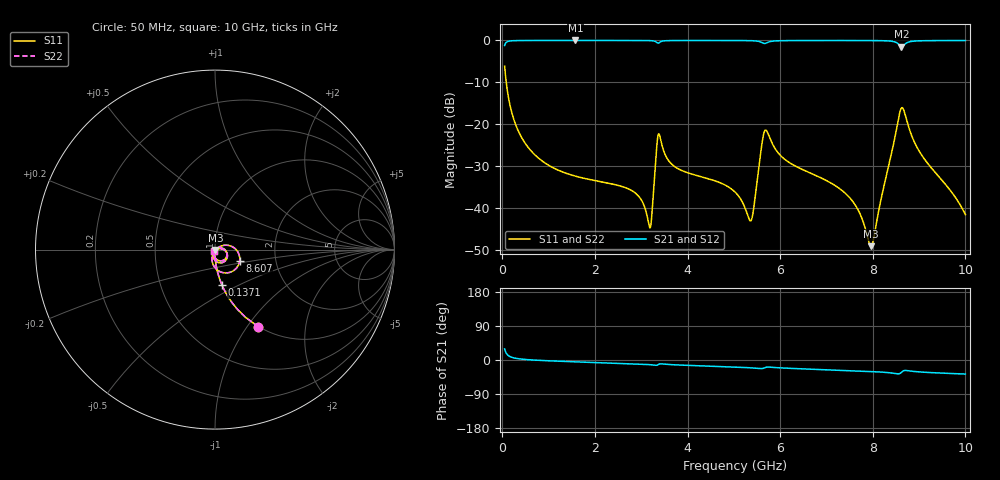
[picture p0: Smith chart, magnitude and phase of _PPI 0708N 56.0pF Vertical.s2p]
! S-Parameter data specifications (vertical orientation):
! Substrate: 40-mil Rogers 3003C, Substrate thickness, H=1.016mm, Dielectric constant, Er=3, Conductor thickness, T_mtl=0.043mm, Loss Tangent, Tand=0.003
! PCB Mounting Pad Footprint: Pad width, PadW=2.54mm , Pad length, PadL=0.51mm , Pad gap, PadG (edge-to-edge)=0.71mm , Reference planes=1.73mm apart
! Created Tue Jan 16 08:53:47 2018
# GHz S MA R 50
! 2 Port Network Data from SP1.SP block
! freq  magS11  angS11  magS21  angS21  magS12  angS12  magS22  angS22
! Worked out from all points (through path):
!   801 points, 50 MHz to 10 GHz, reference 50 ohm
!   highest |S21| = -0.01 dB at 1.58 GHz (marker M1); lowest = -1.5 dB at 8.619 GHz (marker M2)
!   group delay of S21, straight-line fit = 11.2 ps
!   lowest |S11| = -49.1 dB at 7.96 GHz (marker M3), VSWR 1.01, Z = 50.3 - j0.233 ohm
!   |S11| at or under -10 dB: 85.18 MHz to end of sweep
!   |S22| runs from -49.1 to -6.1 dB; largest |S21 - S12| = 0
!   S11 on the Smith chart (normalised r, x): 50 MHz: 1.00, -1.13; 137.1 MHz: 1.00, -0.41; 8.607 GHz: 1.31, -0.18; 10 GHz: 0.99, -0.02
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0.05  0.4931 -60.6  0.8698 29.3  0.8698 29.3  0.4931 -60.6
0.1370625  0.2029 -78.8  0.979 11.2  0.979 11.2  0.2029 -78.8
0.59725  0.04988 -89.2  0.9985 0.5  0.9985 0.5  0.04988 -89.2
1.579813  0.02404 -93.8  0.9992 -4.8  0.9992 -4.8  0.02404 -93.8
1.716625  0.02299 -94.3  0.9992 -5.4  0.9992 -5.4  0.02299 -94.3
2.823562  0.01581 -96.7  0.9988 -10.2  0.9988 -10.2  0.01581 -96.7
3.171813  0.006086 -56.8  0.9955 -12.2  0.9955 -12.2  0.006086 -56.8
3.221563  0.007358 -5.1  0.9926 -12.7  0.9926 -12.7  0.007358 -5.1
3.370812  0.07653 -32.9  0.9282 -11.6  0.9282 -11.6  0.07653 -32.9
3.743937  0.03066 -98.8  0.9972 -12.9  0.9972 -12.9  0.03066 -98.8
5.025  0.01555 -101.2  0.9976 -18.6  0.9976 -18.6  0.01555 -101.2
5.37325  0.00711 -39.8  0.9931 -20.7  0.9931 -20.7  0.00711 -39.8
5.609563  0.06007 -8.1  0.9415 -22.6  0.9415 -22.6  0.06007 -8.1
5.696625  0.08487 -54.6  0.9293 -19.2  0.9293 -19.2  0.08487 -54.6
6.691625  0.02559 -109.7  0.9974 -24.3  0.9974 -24.3  0.02559 -109.7
7.524938  0.01284 -108.6  0.9975 -28.1  0.9975 -28.1  0.01284 -108.6
7.96025  0.003512 -41.2  0.9962 -30.3  0.9962 -30.3  0.003512 -41.2
8.345812  0.03213 31.8  0.9858 -33.4  0.9858 -33.4  0.03213 31.8
8.607  0.1523 -25.5  0.8488 -34.0  0.8488 -34.0  0.1523 -25.5
8.619438  0.1566 -33.1  0.843 -32.7  0.843 -32.7  0.1566 -33.1
9.017437  0.04626 -110.4  0.9897 -31.5  0.9897 -31.5  0.04626 -110.4
10  0.008351 -110.7  0.9972 -37.1  0.9972 -37.1  0.008351 -110.7
